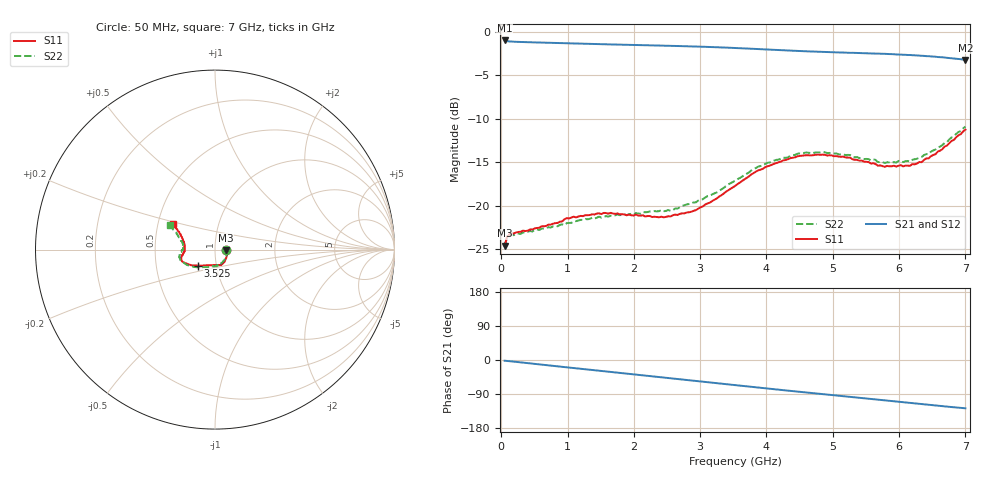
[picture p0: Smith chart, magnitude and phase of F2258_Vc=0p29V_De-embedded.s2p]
! Integrated Device Technology
! Corporate Headquarters
! 6024 Silver Creek Valley Road
! San Jose, CA 95138  USA
! Phone:  1-408-284-8200
! Toll Free:  1-800-223-1366
! Webpage:  http://www.idt.com/
! Timing and RF Division
! 515 Groton Road, Suite 102
! Westford, MA 01886-6024
! Device:  F2258
! Description: Voltage Variable RF Attenuator
! Frequency:  50.0 -  6000.00 MHz
! Package:  3x3 mm Thin QFN Plastic Package: 16 pin
! Ports:  2 RF, 2 DC
!  Pin  1  = NC
!  Pin  2  = NC
!  Pin  3  = RF2  = Port 2
!  Pin  4  = GND
!  Pin  5  = Vdd
!  Pin  6  = NC
!  Pin  7  = VCTRL
!  Pin  8  = NC
!  Pin  9  = GND
!  Pin 10  = RF1  = Port 1
!  Pin 11  = NC
!  Pin 12  = NC
!  Pin 13  = NC
!  Pin 14  = NC
!  Pin 15  = NC
!  Pin 16  = NC
! Vcntrl:  0.290 Volts
! Vdd:  +3.300 Volts
! Current:  1.085 mA
! Data:  The device was measured on a the F2258 evaluation board which has
!  individual transmission lines to the RF pins.  Data was collected
!  using a calibrated network analyzer.  The evaluation board was
!  de-embedded using a TRL calibration technique.
!  The reference plane is the edge of the package pin.
! Misc:  SN 10
!  Action Tracker AT0285
! Date Measured:  2014-12-10
! Date:  2016-01-13  MJV
! Note:
!  Integrated Device Technology supplies this data as a sample of measured
!  data at the package pin for this product.  Your particular data for this
!  product may vary.
!  Data was taken at 25 degrees C.
!  Integrated Device Technology reserves the right to change this data at anytime.
!Freq_(GHz)  S11M_(dB)  S11P_(deg)  S21M_(dB)  S21P_(deg)  S12M_(dB)  S12P_(deg)  S22M_(dB)  S22P_(deg)
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# GHz S dB R 50
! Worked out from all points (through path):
!   201 points, 50 MHz to 7 GHz, reference 50 ohm
!   highest |S21| = -0.97 dB at 50 MHz (marker M1); lowest = -3.2 dB at 7 GHz (marker M2)
!   group delay of S21, straight-line fit = 50.5 ps
!   lowest |S11| = -24.6 dB at 50 MHz (marker M3), VSWR 1.13, Z = 56.3 - j0.395 ohm
!   |S11| at or under -10 dB: start of sweep to end of sweep
!   |S22| runs from -24.6 to -10.9 dB; largest |S21 - S12| = 0.00046
!   S11 on the Smith chart (normalised r, x): 50 MHz: 1.13, -0.01; 3.525 GHz: 0.81, -0.15; 7 GHz: 0.60, +0.19
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0.05  -24.59 -3.4  -0.97 -1.9  -0.97 -1.9  -24.64 -3.0
0.08475  -23.63 -5.8  -1.05 -2.5  -1.05 -2.5  -23.72 -5.3
0.15425  -23.15 -9.0  -1.10 -3.6  -1.10 -3.6  -23.34 -9.3
0.71025  -22.17 -36.4  -1.24 -14.1  -1.24 -14.1  -22.46 -38.1
0.98825  -21.42 -50.1  -1.29 -19.3  -1.29 -19.3  -21.99 -54.1
1.2315  -21.19 -58.3  -1.35 -23.8  -1.35 -23.8  -21.62 -63.1
1.6485  -20.81 -69.9  -1.43 -31.4  -1.43 -31.4  -21.14 -76.1
2.37825  -21.32 -91.1  -1.56 -44.8  -1.56 -44.8  -20.62 -93.8
2.552  -21.23 -97.0  -1.59 -48.0  -1.59 -48.0  -20.58 -99.1
2.93425  -20.50 -113.7  -1.67 -55.1  -1.67 -55.1  -19.60 -112.5
3.525  -17.72 -136.8  -1.84 -66.2  -1.84 -66.2  -17.12 -135.2
4.0115  -15.46 -150.6  -2.02 -75.2  -2.02 -75.2  -15.06 -150.7
4.46325  -14.31 -159.1  -2.18 -83.4  -2.18 -83.4  -14.02 -161.9
4.7065  -14.18 -162.4  -2.25 -87.7  -2.25 -87.7  -13.91 -166.1
5.15825  -14.34 -167.8  -2.37 -95.6  -2.37 -95.6  -14.09 -173.0
5.61  -15.11 -174.6  -2.47 -103.5  -2.48 -103.5  -14.65 -179.1
5.6795  -15.39 -176.1  -2.49 -104.6  -2.49 -104.6  -14.97 -179.6
5.85325  -15.45 179.7  -2.54 -107.8  -2.54 -107.8  -15.00 175.8
6.166  -15.39 171.9  -2.65 -113.4  -2.65 -113.4  -14.91 169.9
6.33975  -14.98 165.5  -2.73 -116.5  -2.73 -116.5  -14.37 165.5
6.722  -13.06 153.8  -2.96 -123.1  -2.97 -123.1  -12.67 156.5
7  -11.24 148.3  -3.21 -127.4  -3.21 -127.4  -10.89 151.5
